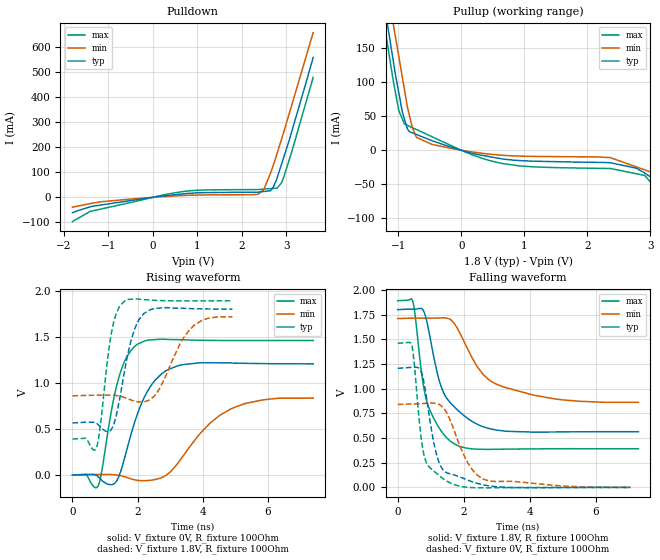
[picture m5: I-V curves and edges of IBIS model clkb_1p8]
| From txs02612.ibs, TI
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|   clkb_1p8 Model
[Model]   clkb_1p8
Model_type   Output
Polarity   Non-Inverting
Vmeas = 0.9
Vref = 0.9
Cref = 15pF
Rref = 100
|   typ   min   max
|   (nom PVT)   (fast PVT)   (slow PVT)
|C_comp from frequency sweep method (F=60MHz)
C_comp   6.218e-12   6.206e-12   6.378e-12
|ON state : BUFFER OUTPUT TURNED HIGH
|C_comp   6.218e-12   6.206e-12   6.378e-12
|OFF state: BUFFER OUTPUT TURNED LOW
|C_comp   5.492e-12   5.379e-12   5.693e-12
|C_comp from LC tank measurement(L=1nH)
|Resonant Frequency(Hz)   2.060e+09   2.070e+09   2.040e+09
|C_comp   5.975e-12   5.917e-12   6.093e-12
|ON state : BUFFER OUTPUT TURNED HIGH
|Resonant Frequency(Hz)   2.060e+09   2.070e+09   2.040e+09
|C_comp   5.975e-12   5.917e-12   6.093e-12
|OFF state: BUFFER OUTPUT TURNED LOW
|Resonant Frequency(Hz)   2.190e+09   2.190e+09   2.180e+09
|C_comp   5.287e-12   5.287e-12   5.335e-12
| Where nom  PVT is Nominal Process, 1.8V, 27C
|   Fast PVT is Strong Process,  1.89V, -40C
|   Slow PVT is Weak Process,   1.71V, 125C
[Voltage Range]   1.8   1.71   1.89
|Ambient Temperature   25   85   -40
|Junction Temperature
[Temperature Range]   27   125   -40
[Pullup Reference]   1.8   1.71   1.89
[Pulldown Reference]   0   0   0
[Power Clamp Reference]   1.8   1.71   1.89
[GND Clamp Reference]   0   0   0
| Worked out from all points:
|   slope of the pulldown table from 0 to 0.27 V, typ, clamps not added: 42.1 ohm
|   slope of the pullup table from 0 to 0.27 V, typ, clamps not added: 41.8 ohm
|   falling waveform, V_fixture 1.8V, R_fixture 100Ohm: 20-80 % time 766ps typ, 1.18ns min, 526ps max; typ from 1.8 V to 0.565 V
|   rising waveform, V_fixture 0V, R_fixture 100Ohm: 20-80 % time 758ps typ, 1.3ns min, 515ps max; typ from 0 V to 1.21 V
|   rising waveform, V_fixture 1.8V, R_fixture 100Ohm: 20-80 % time 440ps typ, 720ps min, 318ps max; typ from 0.565 V to 1.8 V
|   falling waveform, V_fixture 0V, R_fixture 100Ohm: 20-80 % time 422ps typ, 686ps min, 300ps max; typ from 1.21 V to 0 V
[Pulldown]
|   Voltage   I(typ)   I(min)   I(max)
-1.8V     -61.7mA    -39.36mA   -96.94mA
-1.4V     -37.94mA   -25.05mA   -56.08mA
563.2mV   11.6mA     6.323mA    20.14mA
1.058V    18.35mA    9.187mA    28.85mA
2.365V    20.8mA     12.34mA    31.17mA
2.491V    23.36mA    31.45mA    32.92mA
2.641V    26.37mA    95.7mA     34.99mA
2.7V      38.75mA    126.5mA    35.81mA
2.792V    78.46mA    176.3mA    37.07mA
2.89V     132.8mA    232.6mA    58.3mA
3.113V    259.5mA    365.5mA    178.4mA
3.6V      559.8mA    659.4mA    480.3mA
[Pullup]
|   Voltage   I(typ)   I(min)   I(max)
-1.8V     576.4mA    620.1mA    551.7mA
-1.227V   217.3mA    270mA      188mA
-1.208V   205.5mA    258.5mA    177mA
-1.151V   172.4mA    223.7mA    143.5mA
-1.081V   131.9mA    185.9mA    102.5mA
-990.4mV  83.51mA    136.8mA    57.91mA
-855mV    31.35mA    63.59mA    36.57mA
-713.1mV  23.15mA    19.03mA    30.5mA
655.8mV   -12.82mA   -7.351mA   -19.43mA
2.362V    -18.29mA   -10.75mA   -26.72mA
2.911V    -33.43mA   -28.76mA   -36.96mA
3.6V      -78.99mA   -51.42mA   -111.2mA
[Ramp]
R_load = 100
|   typ   min   max
dV/dt_r   0.723657/7.58254e-10   0.504276/1.31303e-09   0.875628/5.14426e-10
dV/dt_f   0.740824/7.63705e-10   0.510336/1.18805e-09   0.899149/5.25195e-10
[Falling Waveform]
V_fixture = 1.8V
V_fixture_min = 1.71V
V_fixture_max = 1.89V
R_fixture = 100Ohm
|   Time   V(typ)   V(min)   V(max)
0s        1.8V       1.71V      1.89V
460ps     1.805V     1.714V     1.881V
775ps     1.791V     1.714V     1.038V
955ps     1.562V     1.714V     798.3mV
1.275ns   1.061V     1.716V     592.3mV
1.71ns    816.9mV    1.66V      442mV
2.42ns    637.8mV    1.217V     387.5mV
3ns       580.9mV    1.043V     387.2mV
4.74ns    561.5mV    896.8mV    391.5mV
7.285ns   564.5mV    861.8mV    391.4mV
[Rising Waveform]
V_fixture = 0V
V_fixture_min = 0V
V_fixture_max = 0V
R_fixture = 100Ohm
|   Time   V(typ)   V(min)   V(max)
0s        64.59nV    5.571uV    13nV
785ps     -15.74mV   6.255mV    -118mV
1.365ns   -58.91mV   601.6uV    980mV
1.675ns   283.6mV    -26.15mV   1.287V
2.005ns   672mV      -57.43mV   1.421V
2.545ns   1.032V     -47.65mV   1.47V
3.22ns    1.183V     121.2mV    1.469V
4.225ns   1.219V     563.4mV    1.461V
4.86ns    1.216V     716.4mV    1.459V
7.395ns   1.206V     834mV      1.459V
[Rising Waveform]
V_fixture = 1.8V
V_fixture_min = 1.71V
V_fixture_max = 1.89V
R_fixture = 100Ohm
|   Time   V(typ)   V(min)   V(max)
0s        565.3mV    859.4mV    391.4mV
735ps     562.8mV    866.2mV    295.4mV
830ps     532.9mV    866.7mV    464.4mV
1.2ns     498.7mV    866.5mV    1.548V
1.35ns    655mV      862.3mV    1.756V
1.6ns     1.126V     841.3mV    1.886V
1.915ns   1.589V     801.1mV    1.911V
2.36ns    1.788V     812.9mV    1.899V
3.755ns   1.804V     1.63V      1.889V
4.915ns   1.8V       1.716V     1.89V
[Falling Waveform]
V_fixture = 0V
V_fixture_min = 0V
V_fixture_max = 0V
R_fixture = 100Ohm
|   Time   V(typ)   V(min)   V(max)
0s        1.206V     840.5mV    1.459V
430ps     1.216V     845.4mV    1.435V
495ps     1.217V     845.9mV    1.276V
710ps     1.173V     849.2mV    500.9mV
860ps     936mV      852.3mV    257.7mV
1.135ns   387.4mV    851.1mV    154.3mV
1.46ns    153.3mV    768.8mV    69.75mV
2.115ns   74.7mV     253.2mV    1.985mV
2.605ns   25.99mV    82.96mV    -3.764mV
7.045ns   396.1uV    2.46mV     6.811uV
